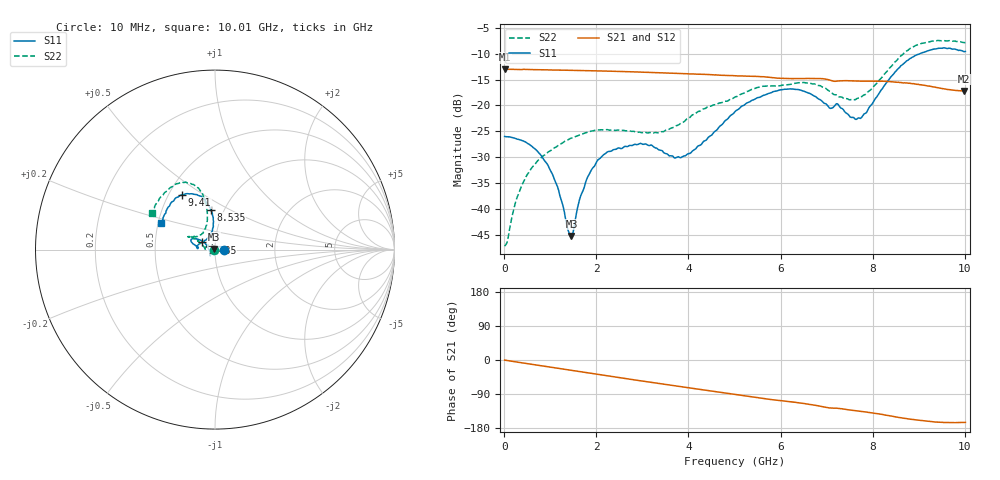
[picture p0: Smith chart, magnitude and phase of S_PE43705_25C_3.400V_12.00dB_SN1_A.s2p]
! Device ID: PE43705
! Serial: 1
! Insertion: A
! Impedance: 50 ohm
! Temp: 25C
! VDD: 3.400V
! Attenuation Step: 12.00dB
#  Hz  S  RI  R  50
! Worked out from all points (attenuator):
!   401 points, 10 MHz to 10.01 GHz, reference 50 ohm
!   highest |S21| = -12.97 dB at 10 MHz (marker M1); lowest = -17.2 dB at 9.985 GHz (marker M2)
!   lowest |S11| = -45.3 dB at 1.46 GHz (marker M3), VSWR 1.01, Z = 49.6 + j0.359 ohm
!   |S11| at or under -10 dB: start of sweep to 9.018 GHz
!   |S22| runs from -47.3 to -7.4 dB; largest |S21 - S12| = 0.0019
!   S11 on the Smith chart (normalised r, x): 10 MHz: 1.11, +0.00; 7.435 GHz: 0.86, +0.07; 8.535 GHz: 0.86, +0.40; 9.41 GHz: 0.58, +0.41; 10.01 GHz: 0.52, +0.17
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1e7  0.05 9.99e-05  0.2247 -0.00101  0.2249 -0.000924  -0.00432 0.000423
2.85e8  0.0465 0.00782  0.2221 -0.0215  0.2222 -0.0214  -0.00525 0.0119
5.35e8  0.0398 0.0142  0.219 -0.0401  0.2191 -0.0399  -0.0102 0.02
1.01e9  0.0181 0.0146  0.2085 -0.0728  0.2085 -0.0726  -0.0271 0.0245
1.385e9  -0.000303 0.00622  0.1969 -0.0964  0.197 -0.0964  -0.0416 0.0206
1.46e9  -0.00407 0.00362  0.1941 -0.101  0.1942 -0.1009  -0.0444 0.0189
1.685e9  -0.0135 -0.00413  0.1854 -0.1141  0.1855 -0.114  -0.0511 0.0141
1.885e9  -0.0207 -0.0108  0.177 -0.1252  0.1771 -0.1249  -0.0556 0.00955
2.21e9  -0.0258 -0.023  0.1618 -0.1417  0.162 -0.1417  -0.0581 0.00239
2.935e9  -0.0278 -0.0323  0.1226 -0.1714  0.1229 -0.1713  -0.0552 0.00217
3.36e9  -0.0253 -0.0272  0.0975 -0.1831  0.0977 -0.1828  -0.0543 0.00582
3.985e9  -0.0339 -0.000529  0.059 -0.1939  0.0592 -0.1936  -0.0708 0.0238
5.01e9  -0.0722 0.0488  -0.00208 -0.194  -0.00177 -0.194  -0.1067 0.0564
5.985e9  -0.1282 0.0598  -0.0538 -0.1753  -0.053 -0.1755  -0.1366 0.0737
6.685e9  -0.1223 0.0317  -0.0863 -0.1607  -0.0864 -0.1605  -0.1451 0.0715
7.435e9  -0.0737 0.0401  -0.1134 -0.1316  -0.1129 -0.132  -0.0821 0.0825
7.785e9  -0.032 0.0731  -0.1242 -0.1189  -0.1236 -0.1194  -0.0578 0.1103
8.36e9  -0.0103 0.1806  -0.1429 -0.0927  -0.1424 -0.0929  -0.0457 0.2247
8.535e9  -0.0249 0.2221  -0.1464 -0.0817  -0.1458 -0.0831  -0.0565 0.272
9.41e9  -0.1848 0.3049  -0.1428 -0.041  -0.1428 -0.0408  -0.2194 0.3654
9.985e9  -0.2918 0.1572  -0.1336 -0.0362  -0.1333 -0.037  -0.3444 0.2142
1.001e10  -0.2987 0.1485  -0.1339 -0.0369  -0.1344 -0.0373  -0.3522 0.2037
